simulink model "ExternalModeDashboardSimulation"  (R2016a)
settings: Solver=FixedStepAuto  StartTime=0.0  StopTime=inf  RelTol=1e-3

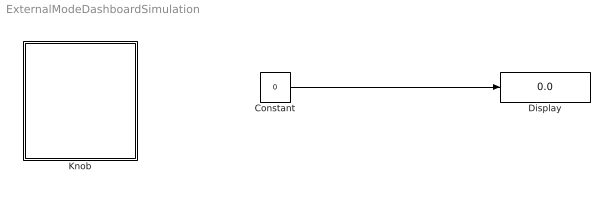
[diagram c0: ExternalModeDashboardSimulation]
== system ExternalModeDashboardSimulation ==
  Constant : Constant  Value=0
  Display : Display
  Knob : Subsystem  DialogController=hmiCreateDDGDialog  IsWebBlock=on
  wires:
  Constant/1 -> Display/1

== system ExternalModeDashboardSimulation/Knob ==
